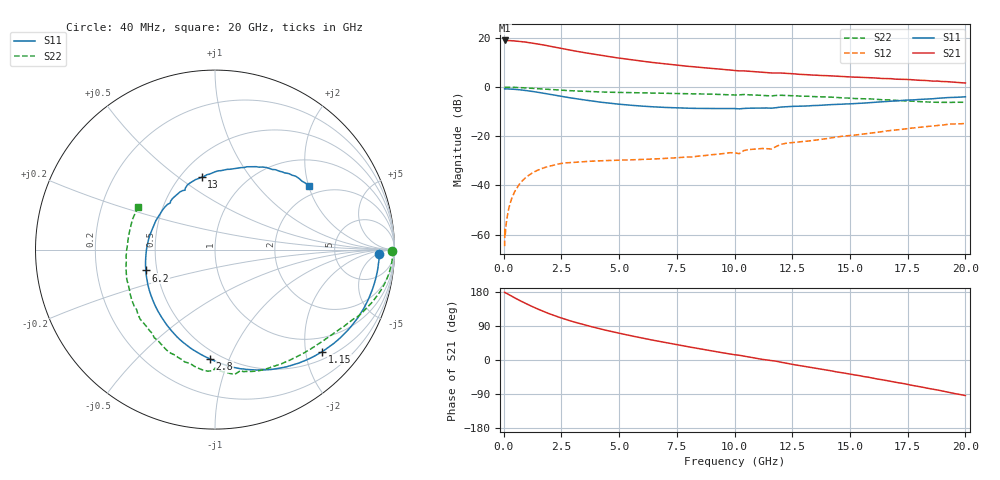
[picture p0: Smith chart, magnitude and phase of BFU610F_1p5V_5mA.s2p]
! Filename:  P:\Prog\Test\Noise\ATS_data\Testdata_Net\SplitFiles\BFU610_2W_A5_HighFreq_1.5V_5mA_D.s2p
! Date/Time: Wed 10/Aug/2011 16:54:14
! BFU610_2W_A5_HighFreq_Bias4_1.5V_1mA_10mA_R.s2p
! MDIF S-parameter v. bias file
! BFU610_2W_A5_HighFreq_1.5V_1mA_10mA
! Date/time Mon Aug 08 13:57:57 2011
! VAR V_out= 1.5001
! VAR I_out= 4.9950
! VAR V_in= 0.9048
! VAR I_in= 0.0411
! Device data file deembeded for feedlines and parallel
! Original file: \SplitFiles\BFU610_2W_A5_HighFreq_1.5V_5mA_R.s2p
! Feed-files: PR003V01_101208_Feed1.s2p, PR003V01_101208_Feed2.s2p
! Parallel-file: PR003V01_101208_Par.s2p
# MHz S MA R 50
!  Freq-MHz  S11-mag  S11-arg  S21-mag  S21-arg  S12-mag  S12-arg  S22-mag  S22-arg
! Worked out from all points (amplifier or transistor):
!   167 points, 40 MHz to 20 GHz, reference 50 ohm
!   highest |S21| = 18.9 dB at 40 MHz (marker M1)
!   |S21| within 3 dB of that: start of sweep to 2.37 GHz
!   unconditionally stable (mu >= 1): 4.128 GHz to end of sweep
!   at 550 MHz: K = 0.09, MSG = 30.0 dB, |S12| = -41.3 dB
!   at 4.2 GHz: K = 1.02, MAG = 20.5 dB, |S12| = -30.0 dB
!   at 20 GHz: K = 1.02, MAG = 7.4 dB, |S12| = -14.8 dB
!   S11 on the Smith chart (normalised r, x): 40 MHz: 21, -6; 1.15 GHz: 0.66, -2.34; 2.8 GHz: 0.44, -0.85; 6.2 GHz: 0.43, -0.12; 13 GHz: 0.63, +0.61; 20 GHz: 1.70, +2.01
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40  0.9156 -1.6  8.826 178.6  0.0005828 88.5  0.9881 -0.3
50  0.9075 -2.2  8.796 178.6  0.001289 87.3  0.9887 -0.5
60  0.9151 -2.1  8.816 177.7  0.0009542 78.8  0.9896 -0.6
180  0.9131 -7.1  8.769 174.1  0.002734 88.2  0.9896 -2.3
360  0.9045 -14.2  8.7 167.9  0.005624 84.5  0.9862 -4.8
750  0.8717 -29.2  8.397 155.3  0.01158 74.6  0.9701 -9.9
1150  0.8247 -43.5  7.927 143.5  0.01688 65.5  0.9468 -14.6
1500  0.778 -55.3  7.451 133.9  0.02064 58.7  0.9243 -18.3
1850  0.7311 -66.3  6.963 125.1  0.02368 52.9  0.9012 -21.7
2250  0.6785 -78.0  6.41 115.9  0.02626 47.9  0.8764 -25.4
2800  0.6102 -92.5  5.725 104.9  0.02904 40.3  0.8446 -29.3
3400  0.5537 -106.9  5.081 94.5  0.03022 36.4  0.8189 -33.5
4000  0.5055 -120.4  4.558 84.9  0.03144 33.5  0.799 -37.4
4600  0.468 -132.7  4.117 76.2  0.03213 31.7  0.7836 -41.3
6200  0.4026 -163.3  3.256 55.5  0.034 31.3  0.7526 -51.9
6800  0.388 -173.8  3.015 48.4  0.03493 32.3  0.7439 -55.8
8600  0.3668 157.0  2.486 28.5  0.03997 37.1  0.7206 -68.2
10200  0.3598 133.9  2.127 12.5  0.04419 41.4  0.6907 -78.4
13000  0.4097 100.3  1.795 -16.5  0.07838 35.5  0.6487 -103.3
13400  0.4196 96.2  1.746 -20.5  0.08212 34.1  0.6386 -107.4
16800  0.5159 63.6  1.474 -56.7  0.1309 14.3  0.5422 -148.7
20000  0.6325 34.2  1.204 -93.9  0.1815 -17.1  0.4889 150.9
